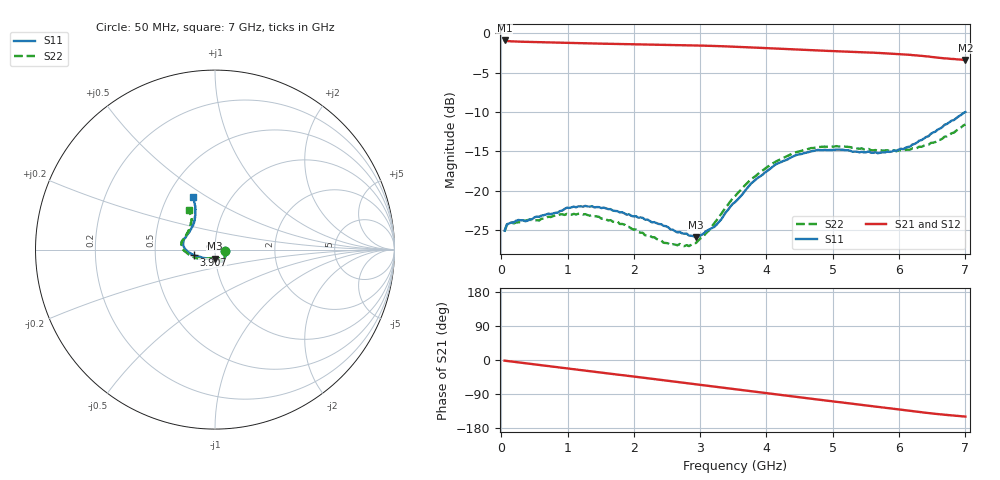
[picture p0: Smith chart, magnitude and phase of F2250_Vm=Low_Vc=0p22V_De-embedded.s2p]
! Integrated Device Technology
! Corporate Headquarters
! 6024 Silver Creek Valley Road
! San Jose, CA 95138  USA
! Phone:  1-408-284-8200
! Toll Free:  1-800-223-1366
! Webpage:  http://www.idt.com/
! Timing and RF Division
! 515 Groton Road, Suite 102
! Westford, MA 01886-6024
! Device:  F2250
! Description: Voltage Variable RF Attenuator
! Frequency:  50.0 -  6000.00 MHz
! Package:  3x3 mm Thin QFN Plastic Package: 16 pin
! Ports:  2 RF, 3 DC
!  Pin  1  = GND
!  Pin  2  = NC
!  Pin  3  = RF1  = Port 1
!  Pin  4  = NC
!  Pin  5  = GND
!  Pin  6  = GND
!  Pin  7  = GND
!  Pin  8  = GND
!  Pin  9  = NC
!  Pin 10  = RF2  = Port 2
!  Pin 11  = NC
!  Pin 12  = GND
!  Pin 13  = GND
!  Pin 14  = VCNTRL
!  Pin 15  = VDD
!  Pin 16  = VMODE
! Vcntrl:  0.220 Volts
! Vmode:  +0.000 Volts
! Vdd:  +3.30  Volts
! Current:  1.107 mA
! Data:  The device was measured on a the F2250 evaluation board which has
!  individual transmission lines to the RF pins.  Data was collected
!  using a calibrated network analyzer.  The evaluation board was
!  de-embedded using a TRL calibration technique.
!  The reference plane is the edge of the package pin.
! Misc:  SN 10
!  Action Tracker AT0258
! Date Measured:  2014-11-26
! Date:  2015-10-15  MJV
! Note:
!  Integrated Device Technology supplies this data as a sample of measured
!  data at the package pin for this product.  Your particular data for this
!  product may vary.
!  Data was taken at 25 degrees C.
!  Integrated Device Technology reserves the right to change this data at anytime.
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# GHz S dB R 50
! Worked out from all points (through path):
!   201 points, 50 MHz to 7 GHz, reference 50 ohm
!   highest |S21| = -0.93 dB at 50 MHz (marker M1); lowest = -3.4 dB at 7 GHz (marker M2)
!   group delay of S21, straight-line fit = 60 ps
!   lowest |S11| = -25.9 dB at 2.934 GHz (marker M3), VSWR 1.11, Z = 49.5 - j5 ohm
!   |S11| at or under -10 dB: start of sweep to end of sweep
!   |S22| runs from -27.1 to -11.6 dB; largest |S21 - S12| = 0.00035
!   S11 on the Smith chart (normalised r, x): 50 MHz: 1.12, -0.02; 3.907 GHz: 0.79, -0.05; 7 GHz: 0.67, +0.43
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0.05  -25.10 -9.7  -0.93 -1.8  -0.93 -1.8  -25.21 -10.1
0.08475  -24.28 -9.6  -1.00 -2.5  -0.99 -2.5  -24.33 -9.4
0.15425  -24.05 -11.9  -1.04 -4.0  -1.04 -4.0  -24.08 -11.1
0.57125  -23.33 -30.0  -1.14 -13.1  -1.14 -13.1  -23.80 -30.4
0.884  -22.60 -45.9  -1.21 -19.9  -1.21 -19.9  -23.03 -46.8
1.2315  -22.04 -56.0  -1.28 -27.4  -1.28 -27.4  -23.04 -59.7
1.75275  -22.61 -62.8  -1.37 -38.4  -1.37 -38.4  -23.93 -66.6
2.37825  -24.25 -63.5  -1.46 -51.8  -1.46 -51.8  -26.26 -67.8
2.552  -24.93 -67.7  -1.49 -55.6  -1.49 -55.6  -26.93 -73.4
2.83  -25.70 -83.2  -1.54 -61.7  -1.54 -61.7  -27.05 -92.7
2.93425  -25.95 -92.3  -1.56 -64.0  -1.56 -64.0  -26.67 -101.5
3.21225  -24.61 -122.0  -1.63 -70.1  -1.63 -70.1  -24.16 -127.5
3.525  -21.47 -148.3  -1.72 -77.1  -1.72 -77.1  -20.71 -146.4
3.76825  -19.10 -161.3  -1.81 -82.5  -1.82 -82.5  -18.56 -156.7
3.90725  -18.18 -165.6  -1.87 -85.5  -1.87 -85.5  -17.66 -162.8
4.1505  -16.62 -173.7  -1.97 -90.8  -1.97 -90.8  -16.27 -171.4
4.7065  -14.97 172.2  -2.18 -102.8  -2.18 -102.8  -14.60 175.6
5.15825  -14.82 161.5  -2.34 -112.5  -2.34 -112.5  -14.36 166.5
5.85325  -15.09 138.4  -2.58 -127.5  -2.59 -127.5  -14.98 151.5
6.166  -14.40 127.5  -2.76 -134.3  -2.76 -134.3  -14.80 142.6
6.444  -13.09 119.3  -2.97 -140.1  -2.97 -140.1  -14.18 133.3
7  -10.01 113.0  -3.41 -149.3  -3.41 -149.3  -11.59 123.9
